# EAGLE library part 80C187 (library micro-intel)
MICROCOMPUTER/PERIPHERAL DEVICE
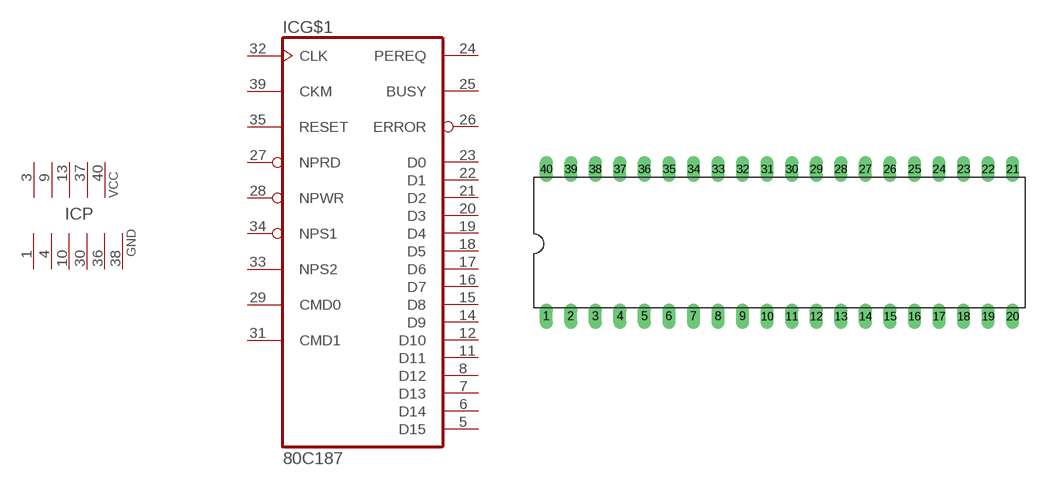
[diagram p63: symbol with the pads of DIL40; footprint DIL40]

Designator prefix IC; gates G$1=80C187 P=5PWR6GND

## 80C187 (OC_FARNELL: unknown; OC_NEWARK: unknown)  [DIL40]
1  P:GND  pwr
3  P:VCC  pwr
4  P:GND  pwr
5  G$1:D15
6  G$1:D14
7  G$1:D13
8  G$1:D12
9  P:VCC  pwr
10  P:GND  pwr
11  G$1:D11
12  G$1:D10
13  P:VCC  pwr
14  G$1:D9
15  G$1:D8
16  G$1:D7
17  G$1:D6
18  G$1:D5
19  G$1:D4
20  G$1:D3
21  G$1:D2
22  G$1:D1
23  G$1:D0
24  G$1:PEREQ  out
25  G$1:BUSY  out
26  G$1:ERROR  out
27  G$1:NPRD  in
28  G$1:NPWR  in
29  G$1:CMD0  in
30  P:GND  pwr
31  G$1:CMD1  in
32  G$1:CLK  in
33  G$1:NPS2  in
34  G$1:NPS1  in
35  G$1:RESET  in
36  P:GND  pwr
37  P:VCC  pwr
38  P:GND  pwr
39  G$1:CKM  in
40  P:VCC  pwr

## Footprint DIL40 (pad centres in mm)
Dual In Line Package
drill 0.813 long: 1 -24.13,-7.62; 2 -21.59,-7.62; 3 -19.05,-7.62; 4 -16.51,-7.62; 5 -13.97,-7.62; 6 -11.43,-7.62; 7 -8.89,-7.62; 8 -6.35,-7.62; 9 -3.81,-7.62; 10 -1.27,-7.62; 11 1.27,-7.62; 12 3.81,-7.62; 13 6.35,-7.62; 14 8.89,-7.62; 15 11.43,-7.62; 16 13.97,-7.62; 17 16.51,-7.62; 18 19.05,-7.62; 19 21.59,-7.62; 20 24.13,-7.62; 21 24.13,7.62; 22 21.59,7.62; 23 19.05,7.62; 24 16.51,7.62; 25 13.97,7.62; 26 11.43,7.62; 27 8.89,7.62; 28 6.35,7.62; 29 3.81,7.62; 30 1.27,7.62; 31 -1.27,7.62; 32 -3.81,7.62; 33 -6.35,7.62; 34 -8.89,7.62; 35 -11.43,7.62; 36 -13.97,7.62; 37 -16.51,7.62; 38 -19.05,7.62; 39 -21.59,7.62; 40 -24.13,7.62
